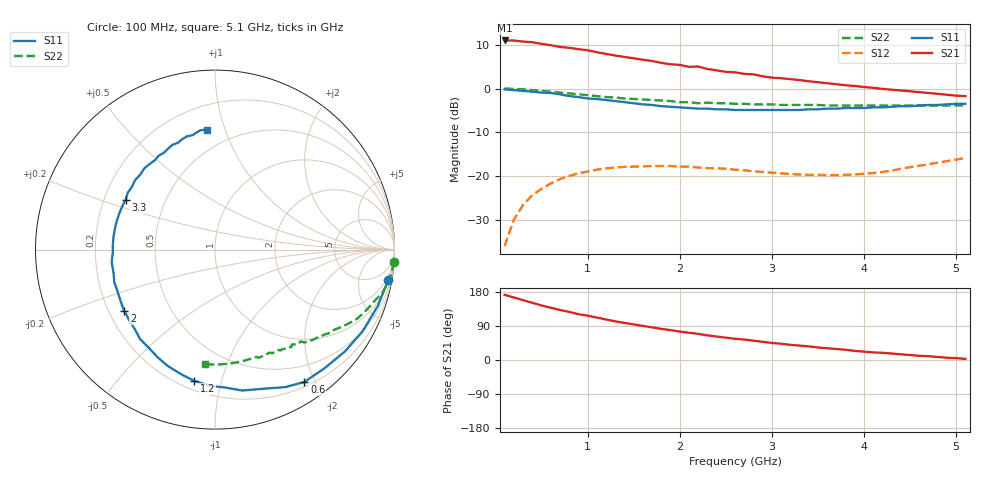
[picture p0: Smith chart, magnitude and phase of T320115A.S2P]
!AT-32011
!S PARAMETERS at Vce=5  V  Ic=1mA.  LAST UPDATED 01-05-95
# ghz s ma r 50
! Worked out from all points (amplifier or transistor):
!   51 points, 100 MHz to 5.1 GHz, reference 50 ohm
!   highest |S21| = 11.0 dB at 100 MHz (marker M1)
!   |S21| within 3 dB of that: start of sweep to 1.182 GHz
!   unconditionally stable (mu >= 1): 2.811 GHz to 5.094 GHz
!   at 900 MHz: K = 0.27, MSG = 14.2 dB, |S12| = -19.3 dB
!   at 2.6 GHz: K = 0.90, MSG = 11.1 dB, |S12| = -18.5 dB
!   at 5.1 GHz: K = 1.00, MSG = 7.0 dB, |S12| = -15.8 dB
!   S11 on the Smith chart (normalised r, x): 100 MHz: 1, -11; 600 MHz: 0.26, -1.85; 1.2 GHz: 0.25, -0.82; 2 GHz: 0.26, -0.29; 3.3 GHz: 0.29, +0.24; 5.1 GHz: 0.36, +0.87
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0.1  0.98 -10.0  3.53 172.0  0.016 83.0  1 -4.0
0.2  0.96 -19.0  3.52 165.0  0.032 78.0  0.99 -8.0
0.4  0.92 -38.0  3.37 151.0  0.061 67.0  0.96 -15.0
0.5  0.9 -47.0  3.23 144.0  0.072 62.0  0.94 -17.0
0.6  0.89 -56.0  3.12 138.0  0.083 57.0  0.92 -20.0
0.7  0.86 -63.0  2.98 132.0  0.093 52.0  0.9 -23.0
0.8  0.82 -71.0  2.91 127.0  0.101 48.0  0.88 -26.0
0.9  0.8 -79.0  2.81 121.0  0.108 45.0  0.86 -28.0
1  0.77 -86.0  2.73 117.0  0.113 41.0  0.84 -30.0
1.2  0.74 -99.0  2.48 107.0  0.123 35.0  0.8 -34.0
1.4  0.7 -112.0  2.29 98.0  0.128 30.0  0.77 -38.0
1.8  0.63 -135.0  1.96 82.0  0.131 21.0  0.73 -44.0
2  0.61 -146.0  1.86 75.0  0.129 18.0  0.7 -47.0
2.1  0.6 -151.0  1.77 72.0  0.129 17.0  0.7 -49.0
2.2  0.59 -158.0  1.78 69.0  0.126 16.0  0.68 -51.0
2.3  0.59 -162.0  1.67 65.0  0.124 15.0  0.69 -52.0
2.6  0.57 -178.0  1.53 56.0  0.119 13.0  0.67 -56.0
3  0.57 164.0  1.33 45.0  0.11 14.0  0.66 -61.0
3.3  0.57 151.0  1.25 38.0  0.105 18.0  0.65 -65.0
3.5  0.58 143.0  1.18 33.0  0.104 21.0  0.65 -68.0
4.3  0.62 115.0  0.97 17.0  0.116 38.0  0.64 -80.0
5.1  0.67 94.0  0.82 3.0  0.162 43.0  0.64 -95.0
